| IBIS file imxrt500_wlcsp141_v1_3.ibs generated by Viper version: 2020.03.16
| This model valid for
| Part Numbers:   Temperature Range:   Package:
| MIMXRT533SFAWCR/MRT533SFAWC   -20C~70C   WLCSP141
| MIMXRT555SFAWCR/MRT555SFAWC   -20C~70C   WLCSP141
| MIMXRT595SFAWCR/MRT595SFAWC   -20C~70C   WLCSP141
[IBIS Ver]   6.0
[Comment Char]   |_char
[File Name]   imxrt500_wlcsp141_v1_3.ibs
[File Rev]   1.2
[Date]   Wed Jan 20 13:09:01 2021
[Source]   NXP Viper 2020.03.16
[Notes]
   Warning 'pullup_ref' Exceeds 15 characters: MIPI_DSI_VDDHA18 was cut to MIPI_DSI_VDDHA1
   Warning 'pullup_ref' Exceeds 15 characters: MIPI_DSI_VDDA_CAP was cut to MIPI_DSI_VDDA_C
[Disclaimer] IMPORTANT NOTICE
  This information is provided on an AS IS basis and without warranty.
  IN NO EVENT SHALL NXP BE LIABLE FOR INCIDENTAL OR CONSEQUENTIAL
  DAMAGES ARISING FROM USE OF THIS INFORMATION. THIS DISCLAIMER OF
  WARRANTY EXTENDS TO THE USER OF THE INFORMATION, AND TO THEIR CUSTOMERS
  OR USERS OF PRODUCTS  AND IS IN LIEU OF ALL WARRANTIES WHETHER EXPRESS,
  IMPLIED, OR STATUTORY, INCLUDING IMPLIED WARRANTIES OF MERCHANTABILITY
  OR FITNESS FOR PARTICULAR PURPOSE.
  NXP does not represent or warrant that the information furnished
  hereunder is free of infringement of any third party patents,
  copyrights, trade secrets, or other intellectual property rights.
  NXP does not represent or warrant that the information is free of
  defect, or that it meets any particular standard, requirements or need
  of the user of the infomation or their customers.
  NXP reserves the right to change the information in this file
  without notice.
   http://www.nxp.com
[Copyright]   (C) Copyright NXP 2004 - 2021, All Rights Reserved.
|   wlcsp141
[Component]   wlcsp141
[Manufacturer]   NXP
[Package]
| variable   typ   min   max
R_pkg   0.23925   0.014244   0.60619
L_pkg   5.000e-10   8.581e-11   1.132e-09
C_pkg   2.827e-13   2.057e-13   4.194e-13
[Pin] signal_name   model_name   R_pin   L_pin   C_pin
A1   GND   GND   NA   NA   NA
A2   GND   GND   NA   NA   NA
A3   VDDIO_0   POWER   NA   NA   NA
A4   PIO3_28   gpio   0.033895  1.664e-10 2.218e-13
A5   PIO1_18   sd_mmc   0.023129  1.489e-10 2.099e-13
A6   PIO1_28   sd_mmc   0.028836  1.664e-10 2.143e-13
A8   PIO4_22   gpiohv   0.024938  1.637e-10 2.155e-13
A10   VDDCORE   POWER   NA   NA   NA
A11   VDD1V8   POWER   NA   NA   NA
A12   GND   GND   NA   NA   NA
B1   VDDIO_0   POWER   NA   NA   NA
B2   VDDCORE   POWER   NA   NA   NA
B3   GND   GND   NA   NA   NA
B4   PIO3_29   gpio   0.16809   3.758e-10 2.547e-13
B5   PIO1_20   sd_mmc   0.14237   3.403e-10 2.413e-13
B6   VDDIO_0   POWER   NA   NA   NA
B7   PIO4_21   gpiohv   0.14757   3.557e-10 2.458e-13
B8   PIO4_20   gpiohv   0.15922   3.802e-10 2.481e-13
B9   PIO4_31   gpiohv   0.11592   2.889e-10 2.312e-13
B10   PIO4_28   gpiohv   0.16285   3.547e-10 2.505e-13
B11   USB0_DM   usbdpdm   0.16865   3.608e-10 2.512e-13
B12   USB0_DP   usbdpdm   0.16604   3.633e-10 2.297e-13
C1   VDDCORE   POWER   NA   NA   NA
C2   PIO1_14   gpio   0.22392   4.546e-10 2.745e-13
C3   VDDCORE   POWER   NA   NA   NA
C4   PIO6_27   gpio   0.26681   5.507e-10 2.927e-13
C5   PIO1_21   sd_mmc   0.29117   6.008e-10 2.988e-13
C6   PIO1_23   sd_mmc   0.28386   5.869e-10 2.956e-13
C7   PIO4_24   gpiohv   0.25631   5.420e-10 2.859e-13
C8   PIO4_27   gpiohv   0.26594   5.592e-10 2.882e-13
C9   PIO4_30   gpiohv   0.23991   5.090e-10 2.795e-13
C10   VDDCORE   POWER   NA   NA   NA
C11   PIO5_8   gpio   0.14389   3.118e-10 2.432e-13
C12   VDDCORE   POWER   NA   NA   NA
D1   PIO1_15   gpio   0.019591  1.058e-10 2.466e-13
D2   PIO1_13   gpio   0.15739   3.485e-10 2.488e-13
D3   PIO1_11   gpio   0.32687   6.527e-10 3.133e-13
D4   PIO1_19   sd_mmc   0.38355   7.596e-10 3.346e-13
D5   PIO1_22   sd_mmc   0.38506   7.629e-10 3.348e-13
D6   PIO4_26   gpiohv   0.40313   7.957e-10 3.415e-13
D7   PIO4_25   gpiohv   0.35386   7.142e-10 3.242e-13
D8   PIO4_29   gpiohv   0.38487   7.679e-10 3.349e-13
D9   PIO5_4   gpio   0.41202   8.075e-10 3.455e-13
D10   USB1_VDD3V3   POWER   NA   NA   NA
D11   VDDIO_1   POWER   NA   NA   NA
E1   VDDIO_0   POWER   NA   NA   NA
E2   PIO1_12   gpio   0.14897   3.279e-10 2.454e-13
E3   PIO0_11   gpio   0.27641   5.684e-10 2.939e-13
E4   PIO0_7   gpio   0.46668   9.011e-10 3.663e-13
E5   VDDIO_3   POWER   NA   NA   NA
E6   VDDCORE   POWER   NA   NA   NA
E7   PIO4_23   gpiohv   0.51273   9.799e-10 3.835e-13
E8   PIO2_24   gpio   0.51832   9.907e-10 3.859e-13
E9   PIO1_6   gpio   0.39134   7.691e-10 3.375e-13
E10   PIO2_27   gpio   0.32943   6.579e-10 3.138e-13
E11   PIO2_26   gpio   0.16462   3.670e-10 2.507e-13
E12   PIO1_5   gpio   0.023523  1.449e-10 2.197e-13
F1   PIO0_10   gpio   0.014451  8.581e-11 2.192e-13
F2   VDDIO_0   POWER   NA   NA   NA
F3   PIO0_9   gpio   0.27108   5.551e-10 2.916e-13
F4   PIO0_4   gpio   0.40619   7.932e-10 3.430e-13
F5   VDD1V8   POWER   NA   NA   NA
F6   VDDCORE   POWER   NA   NA   NA
F7   GND   GND   NA   NA   NA
F8   GND   GND   NA   NA   NA
F9   PIO1_7   gpio   0.42574   8.172e-10 3.501e-13
F10   PIO2_25   gpio   0.31575   6.310e-10 3.085e-13
F11   PIO1_3   gpio   0.25583   5.254e-10 2.859e-13
F12   PIO1_4   gpio   0.10115   2.555e-10 2.276e-13
G1   PIO0_8   gpio   0.014244  8.714e-11 2.199e-13
G2   PIO0_3   gpio   0.16245   3.582e-10 2.503e-13
G3   PIO0_1   gpio   0.3231   6.479e-10 3.116e-13
G4   VDDIO_0   POWER   NA   NA   NA
G5   PIO0_12   gpio   0.60619   1.132e-09 4.194e-13
G6   VDDIO_1   POWER   NA   NA   NA
G7   VDDCORE   POWER   NA   NA   NA
G8   GND   GND   NA   NA   NA
G9   GND   GND   NA   NA   NA
G10   MIPI_DSI_VDD18   POWER   NA   NA   NA
G11   GND   GND   NA   NA   NA
G12   VDDCORE   POWER   NA   NA   NA
H1   GND   GND   NA   NA   NA
H2   PIO0_2   gpio   0.15097   3.338e-10 2.461e-13
H3   PIO0_5   gpio   0.35016   6.962e-10 3.218e-13
H4   PIO0_19   gpio   0.48232   9.234e-10 3.717e-13
H5   VDDIO_1   POWER   NA   NA   NA
H6   PIO0_25   gpio   0.44449   8.107e-10 3.771e-13
H7   GND   GND   NA   NA   NA
H8   MIPI_DSI_D0P   mipi   0.52807   9.813e-10 3.896e-13
H9   MIPI_DSI_D0N   mipi   0.5196   9.727e-10 3.575e-13
H10   GND   GND   NA   NA   NA
H11   MIPI_DSI_CLKP   mipi   0.18818   3.890e-10 2.367e-13
H12   MIPI_DSI_VDD11   POWER   NA   NA   NA
J1   PIO0_0   gpio   0.015425  9.680e-11 2.215e-13
J2   PIO0_13   gpio   0.15482   3.540e-10 2.470e-13
J3   VDDA_ADC1V8   POWER   NA   NA   NA
J4   PIO0_18   gpio   0.41656   8.127e-10 3.469e-13
J5   PIO0_22   gpio   0.34708   6.900e-10 3.210e-13
J6   PIO0_31   gpio   0.33978   6.655e-10 3.305e-13
J7   PIO0_29   gpio   0.35214   6.916e-10 3.218e-13
J8   VSSA   GND   NA   NA   NA
J9   PMIC_MODE1   reset   0.54123   1.028e-09 3.950e-13
J10   RTCXIN   POWER   0.36693   7.171e-10 3.282e-13
J11   MIPI_DSI_VSS   GND   NA   NA   NA
J12   MIPI_DSI_CLKN   mipi   0.18965   3.949e-10 2.601e-13
K1   PIO0_6   gpio   0.017503  1.248e-10 2.057e-13
K2   PIO2_14   gpio   0.13595   3.301e-10 2.388e-13
K3   VSSA   GND   NA   NA   NA
K4   PIO0_15   gpio   0.25365   5.320e-10 2.845e-13
K5   PIO2_31   gpio   0.22566   4.823e-10 2.739e-13
K6   PIO0_14   gpio   0.2298   4.870e-10 2.755e-13
K7   PIO2_30   gpio   0.29778   6.047e-10 3.019e-13
K8   XTALOUT   POWER   0.3695   7.246e-10 3.298e-13
K9   PMIC_IRQ   gpio   0.35274   6.982e-10 3.234e-13
K10   PMIC_MODE0   reset   0.38575   7.502e-10 3.360e-13
K11   RTCXOUT   POWER   0.2364   4.795e-10 2.793e-13
K12   MIPI_DSI_VDDA_CAP   POWER   NA   NA   NA
L1   PIO2_15   gpio   0.018174  1.146e-10 2.071e-13
L2   PIO1_9   gpio   0.14246   3.383e-10 2.181e-13
L3   PIO0_30   gpio   0.16209   3.762e-10 2.493e-13
L4   PIO0_24   gpio   0.17618   3.963e-10 2.549e-13
L5   PIO0_23   gpio   0.15334   3.414e-10 2.463e-13
L6   VDDIO_1   POWER   NA   NA   NA
L7   PIO1_0   gpio   0.18612   4.009e-10 2.591e-13
L8   VDD1V18   POWER   NA   NA   NA
L9   XTALIN   POWER   0.20681   4.257e-10 2.689e-13
L10   VDD_AO1V8   POWER   NA   NA   NA
L11   RESETN   gpio   0.13746   3.028e-10 2.414e-13
L12   VDD1V8   POWER   NA   NA   NA
M1   GND   GND   NA   NA   NA
M2   PIO0_17   gpio   0.025449  1.430e-10 2.261e-13
M3   PIO0_16   gpio   0.024063  1.534e-10 2.181e-13
M4   PIO0_21   gpio   0.023805  1.354e-10 2.218e-13
M5   VDDIO_1   POWER   NA   NA   NA
M6   PIO0_28   gpio   0.022525  1.212e-10 2.200e-13
M7   PIO2_29   gpio   0.01525   9.119e-11 2.088e-13
M8   VDDCORE   POWER   NA   NA   NA
M9   GND   GND   NA   NA   NA
M10   VDD1V8_1   POWER   NA   NA   NA
M11   VDD1V8   POWER   NA   NA   NA
M12   GND   GND   NA   NA   NA
[Pin Mapping]   pulldown_ref   pullup_ref
A1   GND   NC
A2   GND   NC
A3   NC   VDDIO_0
A4   GND   VDDIO_0
A5   GND   VDDIO_0
A6   GND   VDDIO_0
A8   GND   VDDIO_3
A10   NC   VDDCORE
A11   NC   VDD1V8
A12   GND   NC
B1   NC   VDDIO_0
B2   NC   VDDCORE
B3   GND   NC
B4   GND   VDDIO_0
B5   GND   VDDIO_0
B6   NC   VDDIO_0
B7   GND   VDDIO_3
B8   GND   VDDIO_3
B9   GND   VDDIO_3
B10   GND   VDDIO_3
B11   GND   USB1_VDD3V3
B12   GND   USB1_VDD3V3
C1   NC   VDDCORE
C2   GND   VDDIO_0
C3   NC   VDDCORE
C4   GND   VDDIO_0
C5   GND   VDDIO_0
C6   GND   VDDIO_0
C7   GND   VDDIO_3
C8   GND   VDDIO_3
C9   GND   VDDIO_3
C10   NC   VDDCORE
C11   GND   VDDIO_1
C12   NC   VDDCORE
D1   GND   VDDIO_0
D2   GND   VDDIO_0
D3   GND   VDDIO_0
D4   GND   VDDIO_0
D5   GND   VDDIO_0
D6   GND   VDDIO_3
D7   GND   VDDIO_3
D8   GND   VDDIO_3
D9   GND   VDDIO_1
D10   NC   USB1_VDD3V3
D11   NC   VDDIO_1
E1   NC   VDDIO_0
E2   GND   VDDIO_0
E3   GND   VDDIO_0
E4   GND   VDDIO_0
E5   NC   VDDIO_3
E6   NC   VDDCORE
E7   GND   VDDIO_3
E8   GND   VDDIO_1
E9   GND   VDDIO_1
E10   GND   VDDIO_1
E11   GND   VDDIO_1
E12   GND   VDDIO_1
F1   GND   VDDIO_0
F2   NC   VDDIO_0
F3   GND   VDDIO_0
F4   GND   VDDIO_0
F5   NC   VDD1V8
F6   NC   VDDCORE
F7   GND   NC
F8   GND   NC
F9   GND   VDDIO_1
F10   GND   VDDIO_1
F11   GND   VDDIO_1
F12   GND   VDDIO_1
G1   GND   VDDIO_0
G2   GND   VDDIO_0
G3   GND   VDDIO_0
G4   NC   VDDIO_0
G5   GND   VDDIO_0
G6   NC   VDDIO_1
G7   NC   VDDCORE
G8   GND   NC
G9   GND   NC
G10   NC   MIPI_DSI_VDD18
G11   GND   NC
G12   NC   VDDCORE
H1   GND   NC
H2   GND   VDDIO_0
H3   GND   VDDIO_0
H4   GND   VDDIO_1
H5   NC   VDDIO_1
H6   GND   VDDIO_1
H7   GND   NC
H8   GND   MIPI_DSI_VDD18
H9   GND   MIPI_DSI_VDD18
H10   GND   NC
H11   GND   MIPI_DSI_VDD18
H12   NC   MIPI_DSI_VDD11
J1   GND   VDDIO_0
J2   GND   VDDIO_0
J3   NC   VDDA_ADC1V8
J4   GND   VDDIO_1
J5   GND   VDDIO_1
J6   GND   VDDIO_1
J7   GND   VDDIO_1
J8   VSSA   NC
J9   GND   VDD_AO1V8
J10   NC   VDD_AO1V8
J11   GND   NC
J12   GND   MIPI_DSI_VDD18
K1   GND   VDDIO_0
K2   GND   VDDIO_0
K3   VSSA   NC
K4   GND   VDDIO_1
K5   GND   VDDIO_1
K6   GND   VDDIO_1
K7   GND   VDDIO_1
K8   NC   VDD1V8_1
K9   GND   VDD_AO1V8
K10   GND   VDD_AO1V8
K11   NC   VDD_AO1V8
K12   NC   MIPI_DSI_VDDA_C
L1   GND   VDDIO_0
L2   GND   VDDIO_1
L3   GND   VDDIO_1
L4   GND   VDDIO_1
L5   GND   VDDIO_1
L6   NC   VDDIO_1
L7   GND   VDDIO_1
L8   NC   VDD1V18
L9   NC   VDD1V8_1
L10   NC   VDD_AO1V8
L11   GND   VDD_AO1V8
L12   NC   VDD1V8
M1   GND   NC
M2   GND   VDDIO_1
M3   GND   VDDIO_1
M4   GND   VDDIO_1
M5   NC   VDDIO_1
M6   GND   VDDIO_1
M7   GND   VDDIO_1
M8   NC   VDDCORE
M9   GND   NC
M10   NC   VDD1V8_1
M11   NC   VDD1V8
M12   GND   NC
[Diff Pin]  inv_pin  vdiff  tdelay_typ tdelay_min tdelay_max
B11   B12   NA   NA   NA   NA
H8   H9   NA   NA   NA   NA
H11   J12   NA   NA   NA   NA
|*   Model Selector   *
[Model Selector] gpio
io_obe1dse0sre0_lr   5mA current driving capability, w/o slew rate (Low Range Typ: 1.80V, Min: 1.71V, Max: 1.98V)
io_obe1dse0sre1_lr   5mA current driving capability, with slew rate (Low Range Typ: 1.80V, Min: 1.71V, Max: 1.98V)
io_obe1dse1sre0_lr   10mA current driving capability, w/o slew rate (Low Range Typ: 1.80V, Min: 1.71V, Max: 1.98V)
io_obe1dse1sre1_lr   10mA current driving capability, with slew rate (Low Range Typ: 1.80V, Min: 1.71V, Max: 1.98V)
[Model Selector] gpiohv
io_obe1dse0sre0_hr   5mA current driving capability, w/o slew rate (High Range Typ: 3.30V, Min: 3.00V, Max: 3.60V)
io_obe1dse0sre0_lr   5mA current driving capability, w/o slew rate (Low Range Typ: 1.80V, Min: 1.71V, Max: 1.98V)
io_obe1dse0sre0_nr   5mA current driving capability, w/o slew rate (Cont. Range Typ: 3.30V, Min: 2.70V, Max: 3.60V)
io_obe1dse0sre1_hr   5mA current driving capability, with slew rate (High Range Typ: 3.30V, Min: 3.00V, Max: 3.60V)
io_obe1dse0sre1_lr   5mA current driving capability, with slew rate (Low Range Typ: 1.80V, Min: 1.71V, Max: 1.98V)
io_obe1dse0sre1_nr   5mA current driving capability, with slew rate (Cont. Range Typ: 3.30V, Min: 2.70V, Max: 3.60V)
io_obe1dse1sre0_hr   10mA current driving capability, w/o slew rate (High Range Typ: 3.30V, Min: 3.00V, Max: 3.60V)
io_obe1dse1sre0_lr   10mA current driving capability, w/o slew rate (Low Range Typ: 1.80V, Min: 1.71V, Max: 1.98V)
io_obe1dse1sre0_nr   10mA current driving capability, w/o slew rate (Cont. Range Typ: 3.30V, Min: 2.70V, Max: 3.60V)
io_obe1dse1sre1_hr   10mA current driving capability, with slew rate (High Range Typ: 3.30V, Min: 3.00V, Max: 3.60V)
io_obe1dse1sre1_lr   10mA current driving capability, with slew rate (Low Range Typ: 1.80V, Min: 1.71V, Max: 1.98V)
io_obe1dse1sre1_nr   10mA current driving capability, with slew rate (Cont. Range Typ: 3.30V, Min: 2.70V, Max: 3.60V)
[Model Selector] mipi
MIPI_HS   MIPI DSI High Speed Mode
MIPI_LP   MIPI DSI Low Power Mode
[Model Selector] reset
io_rst_obe1dse0sre0_lr   5mA current driving capability, w/o slew rate (Low Range Typ: 1.80V, Min: 1.71V, Max: 1.98V)
io_rst_obe1dse0sre1_lr   5mA current driving capability, with slew rate (Low Range Typ: 1.80V, Min: 1.71V, Max: 1.98V)
io_rst_obe1dse1sre0_lr   10mA current driving capability, w/o slew rate (Low Range Typ: 1.80V, Min: 1.71V, Max: 1.98V)
io_rst_obe1dse1sre1_lr   10mA current driving capability, with slew rate (Low Range Typ: 1.80V, Min: 1.71V, Max: 1.98V)
[Model Selector] sd_mmc
BDPROGSCARUDQP_SDMMC_3V3SF_00_MMC   PSW=0 PDRV=0 MODE=1V8 MMC
BDPROGSCARUDQP_SDMMC_3V3SF_00_SD   PSW=0 PDRV=0 MODE=1V8 SD
BDPROGSCARUDQP_SDMMC_3V3SF_01_MMC   PSW=0 PDRV=1 MODE=1V8 MMC
BDPROGSCARUDQP_SDMMC_3V3SF_01_SD   PSW=0 PDRV=1 MODE=1V8 SD
[Model Selector] usbdpdm
FS_driver   Full Speed USB driver
HS_driver   High Speed USB driver
LS_driver   Low Speed USB driver
fs_device_dm_input   Full Speed Device dm Input
fs_device_dp_input   Full Speed Device dp Input
fs_host_input   Full Speed Host Input
hs_input   High Speed USB Input
ls_host_input   Low  Speed Host Input
| End [Component] wlcsp141
| Models and submodels in the file (30): BDPROGSCARUDQP_SDMMC_3V3SF_00_MMC (I/O), BDPROGSCARUDQP_SDMMC_3V3SF_00_SD (I/O), BDPROGSCARUDQP_SDMMC_3V3SF_01_MMC (I/O), BDPROGSCARUDQP_SDMMC_3V3SF_01_SD (I/O), FS_driver (Output), HS_driver (Output), LS_driver (Output), MIPI_HS (Output), MIPI_LP (I/O), fs_device_dm_input (Input), fs_device_dp_input (Input), fs_host_input (Input), hs_input (Input), io_obe1dse0sre0_hr (I/O), io_obe1dse0sre0_lr (I/O), io_obe1dse0sre0_nr (I/O), io_obe1dse0sre1_hr (I/O), io_obe1dse0sre1_lr (I/O), io_obe1dse0sre1_nr (I/O), io_obe1dse1sre0_hr (I/O), io_obe1dse1sre0_lr (I/O), io_obe1dse1sre0_nr (I/O), io_obe1dse1sre1_hr (I/O), io_obe1dse1sre1_lr (I/O), io_obe1dse1sre1_nr (I/O), io_rst_obe1dse0sre0_lr (I/O), io_rst_obe1dse0sre1_lr (I/O), io_rst_obe1dse1sre0_lr (I/O), io_rst_obe1dse1sre1_lr (I/O), ls_host_input (Input)
